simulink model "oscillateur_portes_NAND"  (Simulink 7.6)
settings: Solver=ode23tb  StartTime=0.0  StopTime=0.01  RelTol=1e-3
libraries: fl_lib x4, elec_lib x3, nesl_utility x2

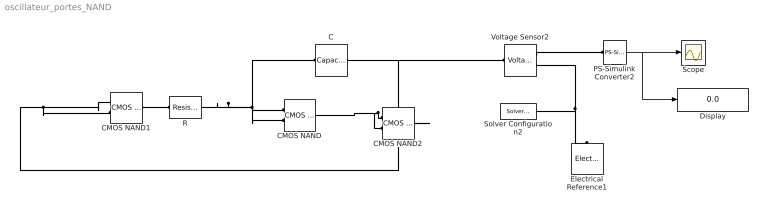
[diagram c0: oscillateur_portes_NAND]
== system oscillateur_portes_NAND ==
  C : fl_lib/Electrical/Electrical Elements/Capacitor  DialogController=NetworkEngine.DynNeDlgSource  SystemSampleTime=-1  c=1e-6 F  v0=5 V  r=1e-6 Ohm  g=0 1/Ohm  i_Log=off  v_Log=off  vc_Log=off  LocalVarNames=|i|v|vc  LocalVarDescs=|i|v|Internal variable for voltage across capacitor term  LocalVarLogging=[0 0 0]
  CMOS NAND : elec_lib/Integrated Circuits/Logic/CMOS NAND  DialogController=NetworkEngine.DynNeDlgSource  SystemSampleTime=-1  V_IL=2 V  V_IH=3 V  C_IN=5 pF  output_type=1  V_OL=0 V  V_OH=5 V  V_CC=5 V  V_meas=5 V  R_OUT=25 Ohm  R_OH=[ 25 250 ] Ohm  I_OH=63 mA  R_OL=[ 30 800 ] Ohm  I_OL=-45 mA  Delay=25 ns  Ron=5 Ohm  Vf=0.6 V  output_state=1  LocalVarLogging=[]
  CMOS NAND1 : elec_lib/Integrated Circuits/Logic/CMOS NAND  DialogController=NetworkEngine.DynNeDlgSource  SystemSampleTime=-1  V_IL=2 V  V_IH=3 V  C_IN=5 pF  output_type=1  V_OL=0 V  V_OH=5 V  V_CC=5 V  V_meas=5 V  R_OUT=25 Ohm  R_OH=[ 25 250 ] Ohm  I_OH=63 mA  R_OL=[ 30 800 ] Ohm  I_OL=-45 mA  Delay=25 ns  Ron=5 Ohm  Vf=0.6 V  output_state=1  LocalVarLogging=[]
  CMOS NAND2 : elec_lib/Integrated Circuits/Logic/CMOS NAND  DialogController=NetworkEngine.DynNeDlgSource  SystemSampleTime=-1  V_IL=2 V  V_IH=3 V  C_IN=5 pF  output_type=1  V_OL=0 V  V_OH=5 V  V_CC=5 V  V_meas=5 V  R_OUT=25 Ohm  R_OH=[ 25 250 ] Ohm  I_OH=63 mA  R_OL=[ 30 800 ] Ohm  I_OL=-45 mA  Delay=25 ns  Ron=5 Ohm  Vf=0.6 V  output_state=1  LocalVarLogging=[]
  Display : Display
  Electrical Reference1 : fl_lib/Electrical/Electrical Elements/Electrical Reference  DialogController=NetworkEngine.DynNeDlgSource  SystemSampleTime=-1  i_Log=off  LocalVarNames=|i  LocalVarDescs=|i  LocalVarLogging=0
  PS-Simulink Converter2 : nesl_utility/PS-Simulink Converter  DialogController=NetworkEngine.DynNeUtilDlgSource  SystemSampleTime=-1  PhysicalDomain=network_engine_domain  LeftPortType=input  RightPortType=output  SubClassName=ps_output  Unit=1  AffineConversion=off
  R : fl_lib/Electrical/Electrical Elements/Resistor  DialogController=NetworkEngine.DynNeDlgSource  SystemSampleTime=-1  R=1 kOhm  i_Log=off  v_Log=off  LocalVarNames=|i|v  LocalVarDescs=|i|v  LocalVarLogging=[0 0]
  Scope : Scope
  Solver Configuration2 : nesl_utility/Solver Configuration  DialogController=NetworkEngine.DynNeUtilDlgSource  SystemSampleTime=-1  PhysicalDomain=network_engine_domain  LeftPortType=input  RightPortType=generic  SubClassName=solver  Accelerate=off  Profile=off  ResidualTolerance=1e-9  MaxNonlinIter=12  MaxModeIter=2  DoFixedCost=off  UseLocalSampling=off  DoDC=off  LinearAlgebra=Sparse  LocalSolverSampleTime=.001  LocalSolverChoice=NE_BACKWARD_EULER_ADVANCER  UseLocalSolver=off
  Voltage Sensor2 : fl_lib/Electrical/Electrical Sensors/Voltage Sensor  DialogController=NetworkEngine.DynNeDlgSource  SystemSampleTime=-1  i1_Log=off  v1_Log=off  LocalVarNames=|i1|v1  LocalVarDescs=|i1|v1  LocalVarLogging=[]
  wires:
  PS-Simulink Converter2/1 -> Scope/1, Display/1
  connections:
  R/RConn1 -- C/RConn1 -- CMOS NAND/LConn1 -- CMOS NAND/LConn2
  Voltage Sensor2/RConn1 -- PS-Simulink Converter2/LConn1
  Voltage Sensor2/RConn2 -- Electrical Reference1/LConn1 -- Solver Configuration2/RConn1
  CMOS NAND2/LConn2 -- CMOS NAND2/LConn1 -- CMOS NAND/RConn1
  CMOS NAND1/RConn1 -- R/LConn1
  C/LConn1 -- CMOS NAND2/RConn1 -- CMOS NAND1/LConn1 -- CMOS NAND1/LConn2 -- Voltage Sensor2/LConn1
